(* Simple derived node - always returns SUCCESS *)
FUNCTION_BLOCK FB_AlwaysSuccess EXTENDS FB_BaseNode

METHOD Tick : E_NodeStatus
Tick := E_NodeStatus.SUCCESS;
eLastStatus := E_NodeStatus.SUCCESS;
SetProgressComplete();
END_METHOD

END_FUNCTION_BLOCK
